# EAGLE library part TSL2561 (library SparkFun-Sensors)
TAOS TSL2561 Digital Luminosity (Light) Sensor The TSL2561 is a light-to-digital converter that transform light intensity to a digital signal output via I2C interface. The device combines one broadband photodiode (visible plus infrared) and one infrared-responding photodiode on a single CMOS integrated circuit capable of providing a near-photopic response over an effective 20-bit dynamic range (16-bit resolution). Two integrating ADCs convert the photodiode currents to a digital output that represents the irradiance measured on each channel. This digital output can be input to a microprocessor where illuminance (ambient light level) in lux is derived using an empirical formula to approximate the human eye response. The TSL2561 device supports a traditional level style interrupt that remains asserted until the firmware clears it. Datasheet SparkFun Products SparkFun Luminosity Sensor Breakout - TSL2561 (SEN-12055)
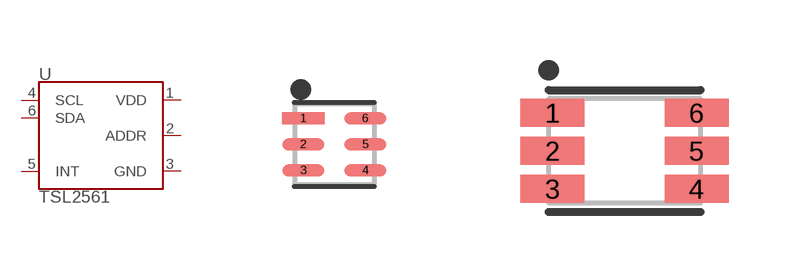
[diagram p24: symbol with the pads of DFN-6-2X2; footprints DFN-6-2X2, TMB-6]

Designator prefix U

## TSL2561FN (PROD_ID: IC-11791)  [DFN-6-2X2]
1  VDD  pwr
2  ADDR  in
3  GND  pwr
4  SCL  in
5  INT  out
6  SDA

## TSL2561T  [TMB-6]
Pads as for DFN-6-2X2

## Footprint DFN-6-2X2 (pad centres in mm)
6-Pin Dual-Flat No-Lead (DFN) (2.0 x 2.0 mm) Datasheet Specifications: Pin Count: 6 Dimensions: 2.0 x 2.0 x 0.65 mm Pitch: 0.65 mm Devices Using: TSL2561
smd 1.05 x 0.3: 1 -0.775,0.65; 2 -0.775,0; 3 -0.775,-0.65; 4 0.775,-0.65; 5 0.775,0; 6 0.775,0.65

## Footprint TMB-6 (pad centres in mm)
6-Pin TMB Datasheet Specifications: Pin Count: 6 Area: 3.8 x 2.6 x 1.35 mm Pitch: 0.9 mm Devices Using: TSL2561
smd 1.6 x 0.7: 1 -1.8,0.95; 2 -1.8,0; 3 -1.8,-0.95; 4 1.8,-0.95; 5 1.8,0; 6 1.8,0.95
